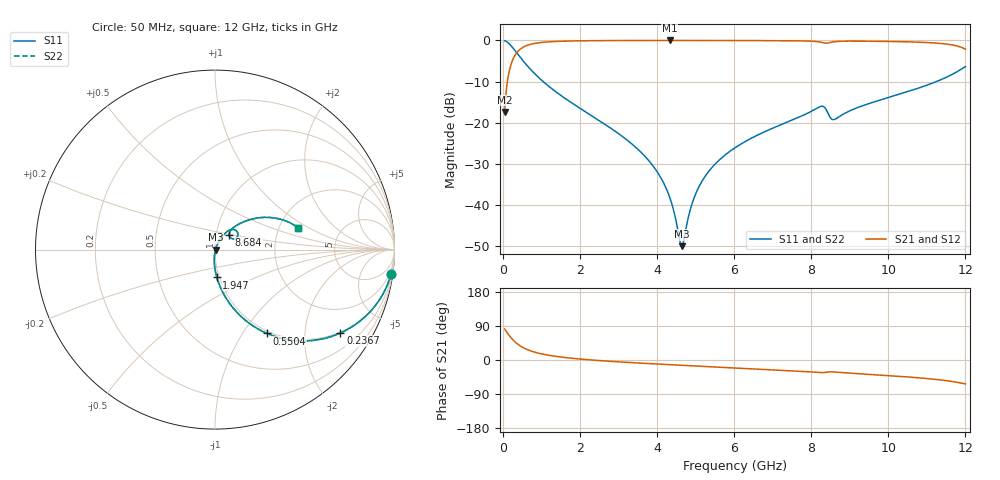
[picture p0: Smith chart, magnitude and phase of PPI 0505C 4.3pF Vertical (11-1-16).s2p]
# GHz S MA R 50
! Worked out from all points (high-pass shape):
!   1601 points, 50 MHz to 12 GHz, reference 50 ohm
!   highest |S21| = -0.03 dB at 4.33 GHz (marker M1); lowest = -17.4 dB at 50 MHz (marker M2)
!   |S21| within 3 dB of the highest: 363.5 MHz to end of sweep
!   lowest |S11| = -50.0 dB at 4.643 GHz (marker M3), VSWR 1.01, Z = 50.3 - j0.0822 ohm
!   |S11| at or under -10 dB: 1.048 GHz to 11.25 GHz (10.2 GHz wide, 166 % of centre)
!   |S22| runs from -50.0 to -0.1 dB; largest |S21 - S12| = 0
!   S11 on the Smith chart (normalised r, x): 50 MHz: 1, -14; 236.7 MHz: 0.96, -3.03; 550.4 MHz: 0.97, -1.29; 1.947 GHz: 0.97, -0.31; 8.684 GHz: 1.16, +0.19; 12 GHz: 2.55, +0.80
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0.05  0.9908 -7.9  0.1351 82.1  0.1351 82.1  0.9908 -7.9
0.1470937  0.9279 -22.3  0.3725 67.7  0.3725 67.7  0.9279 -22.3
0.2367188  0.8393 -33.6  0.5431 56.4  0.5431 56.4  0.8393 -33.6
0.5504062  0.5491 -58.3  0.8347 31.6  0.8347 31.6  0.5491 -58.3
1.028406  0.3221 -74.1  0.9452 15.7  0.9452 15.7  0.3221 -74.1
1.947062  0.1558 -86.2  0.9856 3.1  0.9856 3.1  0.1558 -86.2
2.044156  0.1456 -87.0  0.9871 2.2  0.9871 2.2  0.1456 -87.0
3.33625  0.05586 -94.2  0.9956 -6.9  0.9956 -6.9  0.05586 -94.2
4.038312  0.02402 -93.8  0.9965 -10.8  0.9965 -10.8  0.02402 -93.8
4.329594  0.01246 -88.2  0.9966 -12.3  0.9966 -12.3  0.01246 -88.2
4.643281  0.003165 -15.0  0.9965 -14.0  0.9965 -14.0  0.003165 -15.0
4.912156  0.01041 56.3  0.9964 -15.3  0.9964 -15.3  0.01041 56.3
5.136219  0.01829 62.9  0.9961 -16.5  0.9961 -16.5  0.01829 62.9
5.502187  0.03118 65.2  0.9956 -18.3  0.9956 -18.3  0.03118 65.2
6.025  0.04957 64.7  0.9945 -20.9  0.9945 -20.9  0.04957 64.7
8.019156  0.1386 52.4  0.9759 -31.8  0.9759 -31.8  0.1386 52.4
8.2955  0.1583 38.7  0.9391 -33.3  0.9391 -33.3  0.1583 38.7
8.5345  0.1103 35.0  0.9497 -31.1  0.9497 -31.1  0.1103 35.0
8.683875  0.1146 46.2  0.97 -32.2  0.97 -32.2  0.1146 46.2
10.01331  0.2028 46.1  0.9691 -41.2  0.9691 -41.2  0.2028 46.1
11.25313  0.3163 34.4  0.9253 -51.4  0.9253 -51.4  0.3163 34.4
12  0.4794 14.7  0.7808 -63.1  0.7808 -63.1  0.4794 14.7
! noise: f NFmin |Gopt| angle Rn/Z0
0.05  0.0005584  0.9148  2.051  0.001444
1.372  0.004943  0.729  4.861  0.003625
2.701  0.008098  0.6832  8.547  0.004926
4.031  0.01097  0.6573  12.26  0.006041
5.36  0.01384  0.6435  15.94  0.007212
6.682  0.01727  0.6454  19.56  0.008973
8.012  0.03318  0.7643  23.54  0.02743
9.341  0.02929  0.702  27.05  0.01824
10.67  0.03777  0.7336  30.67  0.02636
12  0.1214  0.8987  34.91  0.2385
